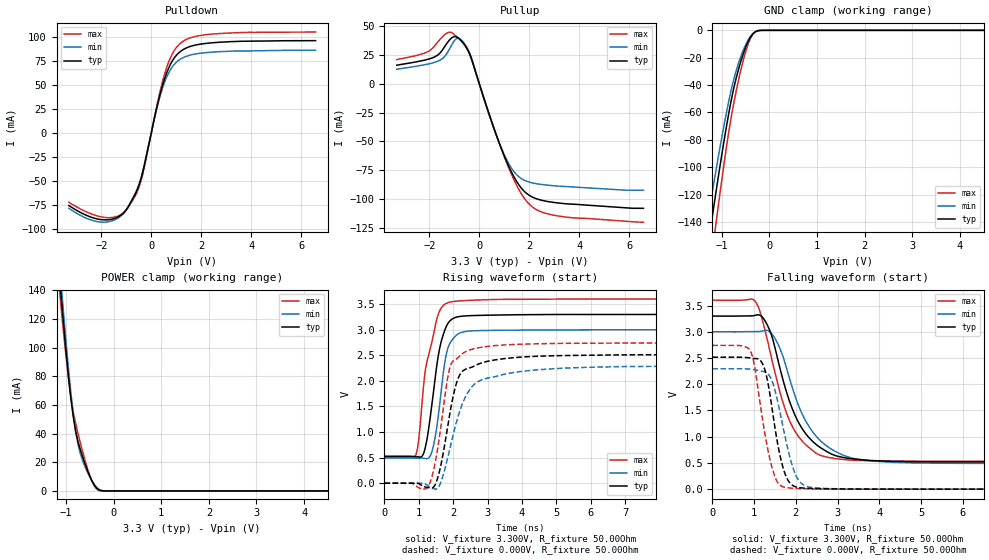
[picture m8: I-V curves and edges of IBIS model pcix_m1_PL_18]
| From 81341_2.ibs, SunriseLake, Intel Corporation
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[Model]   pcix_m1_PL_18
Model_type   I/O
Vinl = 1.155V
Vinh = 1.650V
Vmeas = 1.320V
Vref = 0.000V
Cref = 10.000pF
Rref = 25.000Ohm
|   typ   min   max
C_comp   7.5000pF   6.000pF   9.000pF
[Voltage Range]   3.300V   3.000V   3.600V
[Temperature Range]   60.0   110.0   -5.0
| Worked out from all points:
|   slope of the pulldown table from 0 to 0.495 V, typ, clamps not added: 9.23 ohm
|   slope of the pullup table from 0 to 0.495 V, typ, clamps not added: 15.1 ohm
|   GND clamp passes 1 mA (typ) near -0.30 V on its own axis
|   POWER clamp passes 1 mA (typ) near -0.32 V on its own axis
|   falling waveform, V_fixture 3.300V, R_fixture 50.00Ohm: 20-80 % time 734ps typ, 802ps min, 675ps max; typ from 3.3 V to 0.52 V
|   rising waveform, V_fixture 3.300V, R_fixture 50.00Ohm: 20-80 % time 354ps typ, 295ps min, 410ps max; typ from 0.52 V to 3.3 V
|   rising waveform, V_fixture 0.000V, R_fixture 50.00Ohm: 20-80 % time 438ps typ, 662ps min, 363ps max; typ from 0 V to 2.52 V
|   falling waveform, V_fixture 0.000V, R_fixture 50.00Ohm: 20-80 % time 328ps typ, 394ps min, 346ps max; typ from 2.52 V to 0 V
[Pulldown]
|   Voltage   I(typ)   I(min)   I(max)
-3.3V     -75.85mA   -78.7mA    -72.46mA
-1.9V     -90.82mA   -93.26mA   -88.18mA
-1.35V    -87.97mA   -89.25mA   -87mA
-950mV    -78.15mA   -78.67mA   -78.43mA
-600mV    -61.55mA   -60.75mA   -63.48mA
-400mV    -46.71mA   -45.73mA   -48.86mA
200mV     24.34mA    23.51mA    25.86mA
500mV     54.05mA    50.86mA    58.53mA
850mV     75.7mA     69.47mA    83.06mA
1.25V     86.74mA    78.44mA    95.43mA
2.65V     94.7mA     84.86mA    103.8mA
6.575V    96.49mA    86.43mA    105.5mA
[GND Clamp]
|   Voltage   I(typ)   I(min)   I(max)
-3.3V     -632.5mA   -564.4mA   -725.5mA
-1.325V   -165.6mA   -144.4mA   -196mA
-1.3V     -159.5mA   -139mA     -189mA
-1.25V    -147.6mA   -128.4mA   -175.3mA
-1.2V     -135.8mA   -118mA     -161.6mA
-1.125V   -118.5mA   -102.6mA   -141.4mA
-850mV    -59.64mA   -50.8mA    -72.97mA
-650mV    -28.41mA   -23.93mA   -36.31mA
-450mV    -8.219mA   -7.112mA   -10.14mA
-350mV    -2.584mA   -2.413mA   -2.802mA
-250mV    -331.3uA   -398.2uA   -220.5uA
6.575V    0A         0A         0A
[Pullup]
|   Voltage   I(typ)   I(min)   I(max)
-3.3V     15.92mA    12.41mA    20.73mA
-1.8V     22.94mA    18.3mA     32.25mA
-1.4V     31.41mA    23.06mA    41.9mA
-1.1V     39.58mA    33.46mA    44.16mA
-850mV    39.6mA     39.25mA    39.56mA
-500mV    30.68mA    31.46mA    30.48mA
500mV     -33.06mA   -33.66mA   -32.79mA
1V        -62.31mA   -61.41mA   -62.94mA
1.45V     -82.87mA   -77.62mA   -85.85mA
2V        -96.48mA   -85.07mA   -104.1mA
3.2V      -103.2mA   -88.64mA   -114.5mA
6.575V    -107.7mA   -92.16mA   -119.7mA
[POWER Clamp]
|   Voltage   I(typ)   I(min)   I(max)
-3.3V     1.109A     1.089A     1.13A
-1.15V    154.7mA    163.7mA    144.9mA
-1.1V     134.6mA    143.1mA    126.5mA
-1.05V    115.4mA    123.1mA    109.5mA
-900mV    64.86mA    68.99mA    65.55mA
-800mV    41.99mA    41.86mA    47.4mA
-750mV    34.63mA    32.54mA    40.32mA
-650mV    23.51mA    20.95mA    27.23mA
-500mV    10.16mA    9.585mA    10.63mA
-400mV    3.792mA    4.116mA    3.102mA
-300mV    590.1uA    959uA      205.5uA
6.575V    0A         0A         0A
[Ramp]
R_load = 50.00Ohm
|   typ   min   max
dV/dt_r   1.509V/437.005ps   1.377V/660.837ps   1.645V/362.123ps
dV/dt_f   1.668V/733.982ps   1.505V/801.350ps   1.841V/673.888ps
[Falling Waveform]
V_fixture = 3.300V
V_fixture_min = 3.000V
V_fixture_max = 3.600V
R_fixture = 50.00Ohm
|   Time   V(typ)   V(min)   V(max)
0s        3.3V       3V         3.6V
1.04ns    3.317V     3.005V     3.566V
1.39ns    2.996V     2.99V      2.593V
1.63ns    2.27V      2.662V     1.82V
1.83ns    1.719V     2.16V      1.342V
2.19ns    1.107V     1.37V      883.1mV
2.58ns    796.6mV    930.4mV    647.7mV
3.15ns    601.8mV    642mV      564.5mV
3.88ns    543.1mV    533.5mV    538.8mV
10.3ns    519.6mV    491.1mV    531.7mV
[Rising Waveform]
V_fixture = 3.300V
V_fixture_min = 3.000V
V_fixture_max = 3.600V
R_fixture = 50.00Ohm
|   Time   V(typ)   V(min)   V(max)
0s        519.6mV    491.1mV    531.7mV
910ps     519.8mV    490.7mV    551.7mV
1ns       513.9mV    490.9mV    863.6mV
1.13ns    569.4mV    488.9mV    1.84V
1.43ns    1.797V     745.3mV    2.916V
1.61ns    2.644V     1.551V     3.373V
1.82ns    3.091V     2.575V     3.521V
2.1ns     3.247V     2.897V     3.559V
2.54ns    3.277V     2.978V     3.577V
10.3ns    3.3V       3V         3.6V
[Rising Waveform]
V_fixture = 0.000V
V_fixture_min = 0.000V
V_fixture_max = 0.000V
R_fixture = 50.00Ohm
|   Time   V(typ)   V(min)   V(max)
0s        523.3nV    3.089uV    38.91nV
1.28ns    -85.81mV   -52.3mV    -62.62mV
1.55ns    104mV      -95.74mV   682.5mV
1.81ns    979.3mV    410.8mV    1.934V
1.91ns    1.385V     690.4mV    2.273V
2.15ns    2.058V     1.32V      2.458V
2.43ns    2.245V     1.776V     2.593V
2.87ns    2.361V     2.031V     2.663V
4.35ns    2.479V     2.211V     2.724V
10.3ns    2.515V     2.296V     2.741V
[Falling Waveform]
V_fixture = 0.000V
V_fixture_min = 0.000V
V_fixture_max = 0.000V
R_fixture = 50.00Ohm
|   Time   V(typ)   V(min)   V(max)
0s        2.515V     2.296V     2.741V
900ps     2.502V     2.288V     2.65V
1.01ns    2.49V      2.276V     2.342V
1.18ns    2.421V     2.248V     1.444V
1.31ns    2.109V     2.214V     830.9mV
1.45ns    1.432V     2.018V     357.1mV
1.69ns    419.1mV    1.192V     45.11mV
2ns       43.18mV    262.8mV    14.73mV
2.35ns    13.93mV    34.96mV    6.51mV
10.3ns    523.3nV    3.089uV    38.91nV
